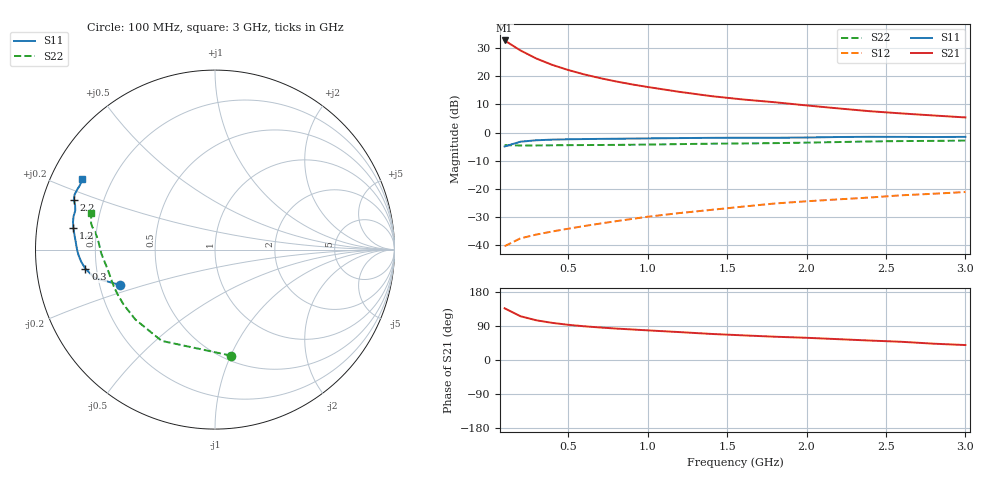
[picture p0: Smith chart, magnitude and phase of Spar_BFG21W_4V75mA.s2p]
! Filename: 475bfg21.001
! Title: BFG21W
! Bias: Vce=4V; Ic=75mA
! Company: NXP Semiconductors NL
! User: Quality&Reliability T&D
! Measure time: 10 Nov 1999 / 11:45:30
#  MHz  S  MA  R 50
! Freq  S11  S21  S12  S22  :
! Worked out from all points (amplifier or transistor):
!   20 points, 100 MHz to 3 GHz, reference 50 ohm
!   highest |S21| = 32.8 dB at 100 MHz (marker M1)
!   |S21| within 3 dB of that: start of sweep to 184.2 MHz
!   unconditionally stable (mu >= 1): 733.6 MHz to end of sweep
!   at 400 MHz: K = 0.82, MSG = 29.6 dB, |S12| = -35.2 dB
!   at 1.2 GHz: K = 1.07, MAG = 19.9 dB, |S12| = -28.6 dB
!   at 3 GHz: K = 1.05, MAG = 11.9 dB, |S12| = -21.1 dB
!   S11 on the Smith chart (normalised r, x): 100 MHz: 0.28, -0.16; 300 MHz: 0.16, -0.07; 1.2 GHz: 0.11, +0.08; 2.2 GHz: 0.09, +0.17; 3 GHz: 0.09, +0.25
100  0.5666 -159.7  43.47 136.4  0.00955 48.5  0.5974 -81.4
200  0.688 -166.7  28.85 115.4  0.01316 45.3  0.5891 -120.3
300  0.73 -171.6  20.72 104.8  0.01537 47.6  0.5904 -138.7
400  0.7489 -174.9  15.99 98.0  0.01743 50.7  0.5944 -149.0
500  0.7599 -177.4  12.96 92.9  0.01951 53.9  0.5975 -155.6
600  0.767 -179.5  10.84 89.0  0.02176 56.8  0.5998 -160.2
700  0.7722 178.7  9.312 85.8  0.02406 59.6  0.6016 -163.8
800  0.7768 177.0  8.13 83.0  0.02653 61.8  0.604 -166.7
900  0.7822 175.4  7.206 80.6  0.02908 63.9  0.6077 -169.3
1000  0.788 173.9  6.468 78.2  0.03186 65.3  0.6123 -171.5
1200  0.7983 171.2  5.304 73.6  0.03703 67.5  0.6237 -175.2
1400  0.8058 169.1  4.451 68.8  0.04219 68.6  0.6341 -178.1
1600  0.8094 166.8  3.879 65.0  0.04825 69.6  0.6406 179.3
1800  0.8083 164.4  3.462 61.5  0.05481 70.2  0.6495 176.5
2000  0.8173 162.4  3.041 58.6  0.06002 71.1  0.6624 173.7
2200  0.8343 160.5  2.692 55.0  0.06488 71.2  0.6785 171.3
2400  0.8403 158.7  2.397 51.3  0.0701 70.6  0.6952 169.5
2600  0.8381 156.8  2.188 48.0  0.07677 69.8  0.7062 167.9
2800  0.8338 154.5  2.013 43.0  0.08172 68.3  0.7117 165.9
3000  0.8387 151.9  1.859 39.4  0.08768 67.5  0.7198 163.3
